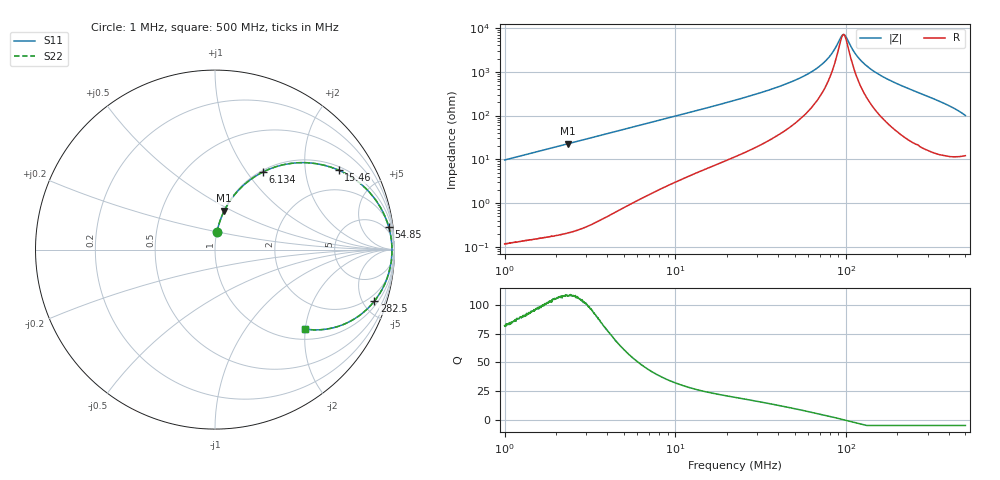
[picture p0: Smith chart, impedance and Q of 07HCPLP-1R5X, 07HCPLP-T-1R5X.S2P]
!s-Parameter Generated by FASTRON Sdn. Bhd.
!FASTRON P/N : 07HCPLP-1R5X, 07HCPLP/T-1R5X
!Keysight Technologies,E4991B,MY54100416,A.01.15
!Date: Tue Feb 03 16:32:25 2026
!Version  : Rev00 Thu Feb 03 16:32:25 2026
!Data & Calibration Information:
!PortZ  Port1:50+j0  Port2:50+j0
!When reading, reference impedance value at option line is always used.
! Remarks : This data is being provided solely for informational purposes.
!Freq	S11	S21	S12	S22
# Hz S dB R 50
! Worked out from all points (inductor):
!   1601 points, 1 MHz to 500 MHz, reference 50 ohm
!   read as one part in series: L = 1.54 uH near 1.032 MHz
!   highest Q = 109 at 2.359 MHz (marker M1), where L = 1.54 uH
!   self-resonance near 96.66 MHz
!   S11 on the Smith chart (normalised r, x): 1 MHz: 1.00, +0.19; 6.134 MHz: 1.02, +1.19; 15.46 MHz: 1.13, +3.03; 54.85 MHz: 3, +15; 282.5 MHz: 1.36, -6.05; 500 MHz: 1.24, -2.00
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1000000  -20.32 83.8  -0.05 -5.5  -0.05 -5.5  -20.32 83.8
2359366  -13.06 76.6  -0.24 -12.8  -0.24 -12.8  -13.06 76.6
2820919  -11.60 74.2  -0.33 -15.2  -0.33 -15.2  -11.60 74.2
6134256  -5.89 58.3  -1.40 -30.5  -1.40 -30.5  -5.89 58.3
7957584  -4.37 51.4  -2.14 -37.2  -2.14 -37.2  -4.37 51.4
1.546086e7  -1.73 32.7  -5.34 -54.9  -5.34 -54.9  -1.73 32.7
2.236068e7  -0.95 23.6  -7.95 -63.5  -7.95 -63.5  -0.95 23.6
3.748322e7  -0.39 13.3  -12.71 -72.4  -12.71 -72.4  -0.39 13.3
5.484648e7  -0.21 7.4  -17.69 -75.7  -17.69 -75.7  -0.21 7.4
6.307767e7  -0.17 5.5  -20.25 -75.6  -20.25 -75.6  -0.17 5.5
7.840424e7  -0.14 2.7  -26.26 -70.2  -26.26 -70.2  -0.14 2.7
8.47377e7  -0.13 1.7  -29.78 -62.5  -29.78 -62.5  -0.13 1.7
9.374216e7  -0.12 0.4  -36.19 -25.6  -36.19 -25.6  -0.12 0.4
9.707707e7  -0.12 -0.1  -37.12 3.6  -37.12 3.6  -0.12 -0.1
1.005306e8  -0.12 -0.5  -35.73 31.6  -35.73 31.6  -0.12 -0.5
1.129546e8  -0.13 -2.0  -28.50 66.4  -28.50 66.4  -0.13 -2.0
1.249575e8  -0.13 -3.3  -24.47 73.4  -24.47 73.4  -0.13 -3.3
1.453951e8  -0.16 -5.4  -20.38 76.3  -20.38 76.3  -0.16 -5.4
1.77937e8  -0.22 -8.5  -16.55 76.0  -16.55 76.0  -0.22 -8.5
2.824894e8  -0.60 -17.9  -10.23 68.7  -10.23 68.7  -0.60 -17.9
3.854345e8  -1.39 -28.0  -6.54 58.2  -6.54 58.2  -1.39 -28.0
5e8  -3.48 -41.4  -3.53 41.7  -3.53 41.7  -3.48 -41.4
